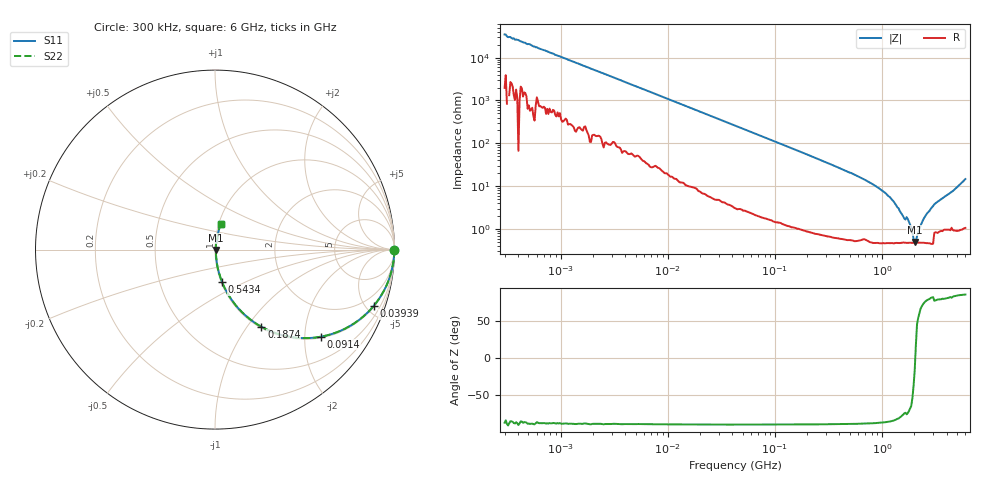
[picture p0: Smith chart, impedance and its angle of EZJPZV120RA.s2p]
!*** S-Parameter ***
!Copyright  (C)  Panasonic Corporation
!Multilaryer Varistors, Chip Type  Port assignments : Series-thru
!  1  o---GGG---o  2
!Parts No. : EZJPZV120RA  GND o---------o GND
# HZ S RI R 50
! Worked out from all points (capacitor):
!   401 points, 300 kHz to 6 GHz, reference 50 ohm
!   read as one part in series: C = 15.7 pF near 315.2 kHz
!   lowest |Z| = 495 mohm at 2.019 GHz (marker M1)
!   series resonance near 2.043 GHz, so ESL is about 390 pH
!   S11 on the Smith chart (normalised r, x): 300 kHz: open; 39.39 MHz: 1.07, -5.59; 91.4 MHz: 1.03, -2.41; 187.4 MHz: 1.02, -1.17; 543.4 MHz: 1.01, -0.38; 6 GHz: 1.02, +0.29
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300000  0.9998 -0.00288  0.000172 0.00288  0.000172 0.00288  0.9998 -0.00288
1575955  0.9993 -0.0149  0.000679 0.0149  0.000679 0.0149  0.9993 -0.0149
8278779  0.9927 -0.0754  0.00726 0.0754  0.00726 0.0754  0.9927 -0.0754
1.828305e7  0.9706 -0.1616  0.0294 0.1616  0.0294 0.1616  0.9706 -0.1616
3.938932e7  0.8834 -0.3148  0.1166 0.3148  0.1166 0.3148  0.8834 -0.3148
4.348994e7  0.8622 -0.339  0.1378 0.339  0.1378 0.339  0.8622 -0.339
9.140418e7  0.5909 -0.4851  0.4091 0.4851  0.4091 0.4851  0.5909 -0.4851
1.874091e8  0.2581 -0.4298  0.7419 0.4298  0.7419 0.4298  0.2581 -0.4298
2.228737e8  0.1975 -0.3899  0.8025 0.3899  0.8025 0.3899  0.1975 -0.3899
5.434398e8  0.0398 -0.1821  0.9602 0.1821  0.9602 0.1821  0.0398 -0.1821
8.278378e8  0.0163 -0.107  0.9837 0.107  0.9837 0.107  0.0163 -0.107
1.170796e9  0.00779 -0.0557  0.9922 0.0557  0.9922 0.0557  0.00779 -0.0557
1.358303e9  0.00594 -0.0348  0.9941 0.0348  0.9941 0.0348  0.00594 -0.0348
1.57584e9  0.00517 -0.019  0.9948 0.019  0.9948 0.019  0.00517 -0.019
1.783508e9  0.00495 -0.0137  0.995 0.0137  0.995 0.0137  0.00495 -0.0137
1.96918e9  0.00476 -0.00361  0.9952 0.00361  0.9952 0.00361  0.00476 -0.00361
2.018543e9  0.00473 -0.00138  0.9953 0.00138  0.9953 0.00138  0.00473 -0.00138
2.121012e9  0.0048 0.00484  0.9952 -0.00484  0.9952 -0.00484  0.0048 0.00484
2.341819e9  0.00491 0.0127  0.9951 -0.0127  0.9951 -0.0127  0.00491 0.0127
2.522384e9  0.00506 0.019  0.9949 -0.019  0.9949 -0.019  0.00506 0.019
2.999709e9  0.00567 0.0339  0.9943 -0.0339  0.9943 -0.0339  0.00567 0.0339
6e9  0.0307 0.1401  0.9693 -0.1401  0.9693 -0.1401  0.0307 0.1401
